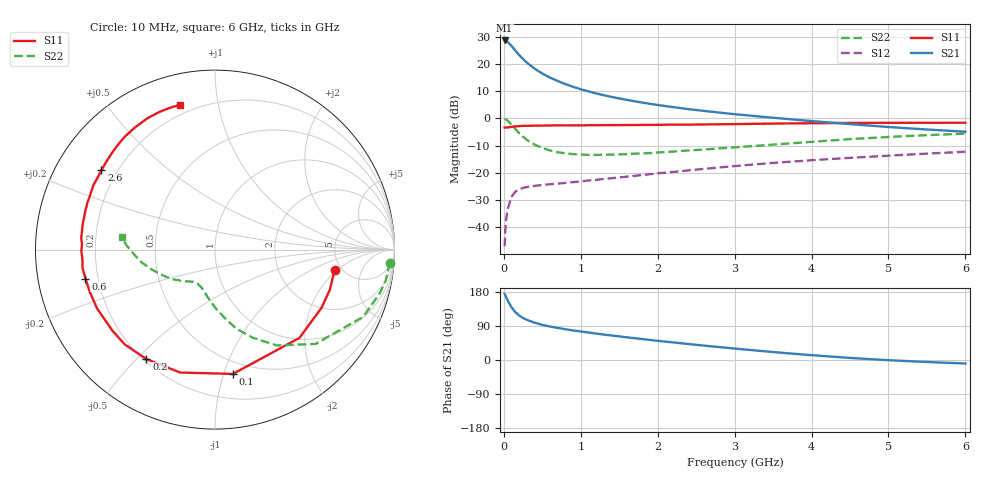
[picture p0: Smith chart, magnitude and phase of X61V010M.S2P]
! SIEMENS Small Signal Semiconductors
! BFP193W
! Si NPN RF Bipolar Junction Transistor in SOT343
! VCE = 1 V  IC = 10 mA
! Common Emitter S-Parameters:  April 1994
# GHz  S  MA  R  50
!  f  S11  S21  S12  S22
! GHz  MAG  ANG  MAG  ANG  MAG  ANG  MAG  ANG
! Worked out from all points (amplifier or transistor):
!   40 points, 10 MHz to 6 GHz, reference 50 ohm
!   highest |S21| = 28.6 dB at 10 MHz (marker M1)
!   |S21| within 3 dB of that: start of sweep to 129.1 MHz
!   unconditionally stable (mu >= 1): 1.217 GHz to 5.47 GHz
!   at 200 MHz: K = 0.23, MSG = 24.6 dB, |S12| = -26.1 dB
!   at 1.5 GHz: K = 1.10, MAG = 12.5 dB, |S12| = -21.7 dB
!   at 6 GHz: K = 0.99, MSG = 3.7 dB, |S12| = -12.3 dB
!   S11 on the Smith chart (normalised r, x): 10 MHz: 4.38, -1.82; 100 MHz: 0.40, -1.07; 200 MHz: 0.21, -0.53; 600 MHz: 0.15, -0.11; 2.6 GHz: 0.14, +0.31; 6 GHz: 0.15, +0.77
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0.01  0.6762 -9.6  26.9 174.4  0.0045 85.1  0.9767 -4.3
0.02  0.6779 -19.3  26.81 170.6  0.0092 80.3  0.9666 -10.3
0.03  0.6764 -28.6  26.49 166.0  0.0139 77.3  0.9492 -15.0
0.05  0.6806 -46.3  25.29 157.1  0.0217 69.5  0.9067 -24.4
0.1  0.6998 -81.8  21.34 139.2  0.0364 54.1  0.7679 -43.2
0.15  0.7118 -105.8  17.55 126.2  0.0451 44.0  0.6354 -57.2
0.2  0.7197 -122.1  14.49 117.3  0.0498 38.1  0.5331 -66.9
0.25  0.7294 -133.6  12.28 110.8  0.0529 34.0  0.4595 -74.5
0.3  0.7285 -141.7  10.49 105.9  0.0548 31.8  0.4008 -80.3
0.4  0.7343 -153.5  8.158 98.4  0.0576 29.1  0.3288 -89.1
0.5  0.7365 -161.4  6.65 92.8  0.0599 28.7  0.2856 -95.6
0.6  0.7394 -167.4  5.59 88.3  0.0616 29.2  0.2571 -101.0
0.8  0.7405 -175.7  4.245 81.2  0.0654 30.9  0.2276 -108.6
1.1  0.748 175.2  3.129 72.5  0.0722 34.4  0.2132 -116.6
1.3  0.7502 170.0  2.655 67.1  0.077 36.6  0.2141 -120.5
1.6  0.754 163.7  2.182 59.8  0.0851 39.4  0.2201 -125.3
2.2  0.7668 152.1  1.608 46.4  0.1039 42.8  0.2454 -134.6
2.6  0.7718 145.1  1.37 38.0  0.118 43.6  0.2673 -140.7
3.2  0.791 135.1  1.123 26.5  0.1404 42.9  0.3073 -149.8
4.5  0.8231 117.2  0.785 5.5  0.1883 37.8  0.4156 -170.2
5.5  0.8286 108.1  0.624 -5.3  0.2251 32.6  0.4913 177.5
6  0.8304 103.7  0.568 -9.2  0.244 30.1  0.5242 172.6
